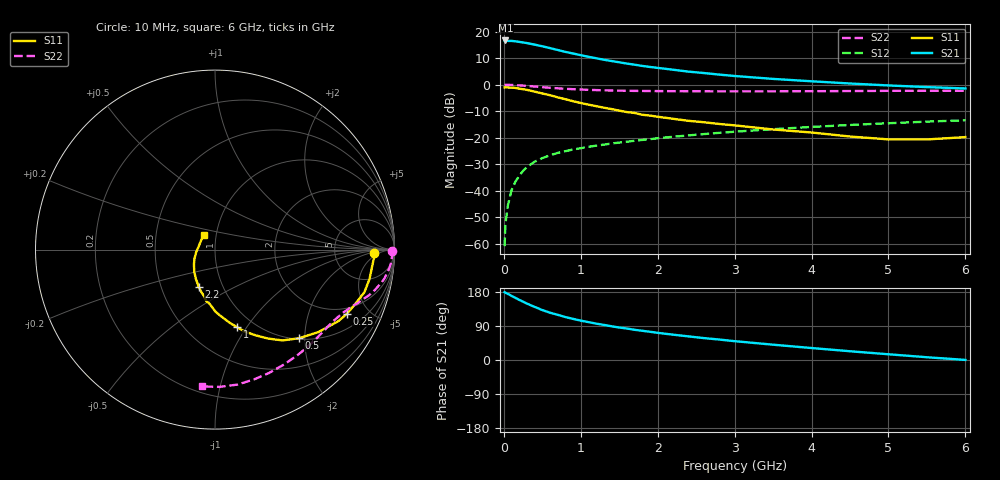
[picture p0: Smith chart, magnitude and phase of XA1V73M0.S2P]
! SIEMENS Discrete & RF Semiconductors
! BFY180
! Si NPN RF Bipolar Junction Transistor in MICRO-X
! VCE = 1.75 V  IC = 3 mA
! Common Emitter S-Parameters:  May  1997
# GHz  S  MA  R  50
!  f  S11  S21  S12  S22
! GHz  MAG  ANG  MAG  ANG  MAG  ANG  MAG  ANG
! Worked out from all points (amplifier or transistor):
!   36 points, 10 MHz to 6 GHz, reference 50 ohm
!   highest |S21| = 16.6 dB at 20 MHz (marker M1)
!   |S21| within 3 dB of that: start of sweep to 616.9 MHz
!   unconditionally stable (mu >= 1): 1.475 GHz to end of sweep
!   at 250 MHz: K = 0.23, MSG = 24.2 dB, |S12| = -32.5 dB
!   at 1.4 GHz: K = 0.98, MSG = 15.6 dB, |S12| = -22.2 dB
!   at 6 GHz: K = 1.15, MAG = 3.6 dB, |S12| = -13.4 dB
!   S11 on the Smith chart (normalised r, x): 10 MHz: 16, -3; 250 MHz: 1.68, -3.62; 500 MHz: 1.02, -1.88; 1 GHz: 0.83, -0.90; 2.2 GHz: 0.77, -0.34; 6 GHz: 0.87, +0.14
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0.01  0.8857 -1.1  6.685 178.9  0.0009 84.1  0.9876 -0.3
0.02  0.8886 -2.3  6.789 177.6  0.0023 92.2  0.99 -0.8
0.05  0.882 -5.2  6.659 174.7  0.0051 86.3  0.9871 -2.0
0.1  0.8764 -10.8  6.661 169.3  0.0102 85.4  0.9842 -4.1
0.2  0.8394 -20.9  6.393 158.7  0.019 77.1  0.9666 -7.9
0.25  0.8176 -25.9  6.21 153.9  0.0237 75.7  0.9575 -9.7
0.3  0.7946 -30.1  6.065 148.9  0.0278 72.8  0.9445 -11.3
0.4  0.7367 -38.6  5.665 140.1  0.0352 68.7  0.9195 -14.1
0.5  0.6806 -46.5  5.27 131.8  0.0411 63.6  0.894 -16.6
0.6  0.6306 -53.4  4.873 124.8  0.0465 61.4  0.8703 -18.5
0.8  0.5296 -64.5  4.131 113.3  0.0556 57.4  0.8329 -21.9
1  0.4495 -74.1  3.58 103.9  0.0633 54.4  0.8064 -24.9
1.1  0.4185 -78.3  3.339 99.9  0.0672 53.5  0.7962 -26.1
1.3  0.367 -85.8  2.941 92.6  0.0739 51.8  0.7805 -28.9
1.5  0.3229 -92.6  2.633 85.7  0.0808 50.4  0.769 -31.6
1.7  0.2921 -99.5  2.371 79.7  0.0873 49.6  0.7601 -34.4
2.2  0.2266 -113.6  1.907 66.8  0.1039 46.6  0.7511 -41.4
2.8  0.1811 -127.9  1.543 54.0  0.1231 42.9  0.7466 -49.7
3.5  0.1425 -145.4  1.28 40.4  0.1445 38.1  0.7467 -59.4
4.5  0.105 -173.4  1.048 23.1  0.1734 30.7  0.7551 -73.3
5.5  0.0924 149.3  0.897 7.3  0.2004 22.7  0.7653 -88.1
6  0.1024 127.8  0.845 0.2  0.2126 18.3  0.7661 -95.5
